(* High speed task. Serial background communication. *)
PROGRAM P_SerialComm_HighSpeed
VAR
	serial_In			AT%I*	: PcComInData;
	serial_Out			AT%Q* 	: PcComOutData;
	KL6_In				AT%I*	: KL6inData5B;
	KL6_Out				AT%Q*	: KL6outData5B;
	serial_ExtStatus 	AT%I*	: WORD;
	serial_ExtCtrl	 	AT%Q* 	: WORD;

	hSerial				: T_HSERIALCTRL;(* Serial connection control handle *)
	fbSerialLineCtrl	: FB_IEC870_SerialLineCtrl := ( Mode := SERIALLINEMODE_PC_COM_PORT(*SERIALLINEMODE_KL6_5B_STANDARD *),
														Baudrate := 19200,
														NoDatabits := 8,
														Parity := PARITY_EVEN,
														Stopbits := 1,
														Handshake := HANDSHAKE_NONE,
														ContinousMode := FALSE );

(* Remove comment brackets if party line mode is used 
	fbPartyLineCtrl : FB_IEC870_PartyLineCtrl := ( eMode := eIEC870_PartylineMode_Ext_On );
	delay 			: TON;
	tRTS_DEALY_ON 	: TIME := T#100ms;
	tRTS_DELAY_OFF 	: TIME := T#100MS;*)
END_VAR

fbSerialLineCtrl(	pComIn := SEL( fbSerialLineCtrl.Mode = SERIALLINEMODE_KL6_5B_STANDARD, ADR( serial_In ), ADR( KL6_In ) ),
					pComOut	:= SEL( fbSerialLineCtrl.Mode = SERIALLINEMODE_KL6_5B_STANDARD, ADR( serial_Out ), ADR( KL6_Out ) ),
					SizeComIn :=  SEL( fbSerialLineCtrl.Mode = SERIALLINEMODE_KL6_5B_STANDARD, SIZEOF( serial_In ), SIZEOF( KL6_In ) ),
					hSerial	 := hSerial );

(* Remove comment brackets if party line mode is used 
fbPartyLineCtrl( hSerial:= hSerial );
IF fbPartyLineCtrl.bRTS <> fbPartyLineCtrl.bCTS THEN
	IF fbPartyLineCtrl.bRTS THEN
		serial_ExtCtrl.1 := TRUE;
		delay( in := TRUE, PT := tRTS_DEALY_ON );
		IF delay.Q THEN
			delay( in := FALSE );
			fbPartyLineCtrl.bCTS := TRUE;
		END_IF
	ELSE
		IF serial_ExtStatus.15 THEN
			delay( in := TRUE, PT := tRTS_DELAY_OFF );
			IF delay.Q THEN
				delay( in := FALSE );
				serial_ExtCtrl.1 := FALSE;
				fbPartyLineCtrl.bCTS := FALSE;
			END_IF
		END_IF
	END_IF
END_IF
*)

END_PROGRAM
